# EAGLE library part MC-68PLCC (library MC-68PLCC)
SOCKET, PLCC, 68 PIN, THRU-HOLE Source: Datasheet
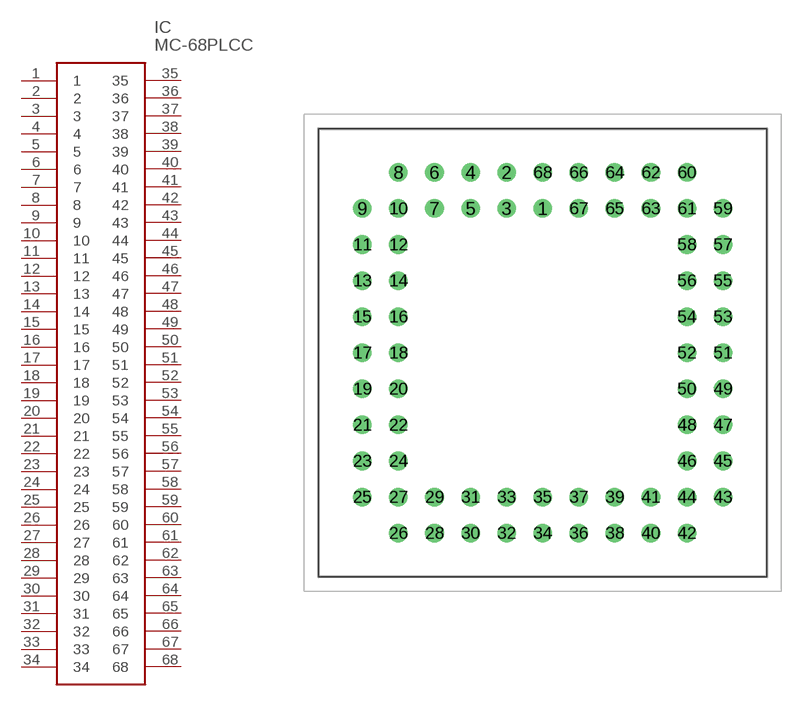
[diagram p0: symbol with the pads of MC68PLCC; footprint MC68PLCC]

Designator prefix IC

## MC-68PLCC (Description: SOCKET, PLCC, 68 PIN, THRU-HOLE; Height: 8.1mm; Manufacturer_Name: MULTICOMP; Manufacturer_Part_Number: MC-68PLCC)  [MC68PLCC]
1  1
2  2
3  3
4  4
5  5
6  6
7  7
8  8
9  9
10  10
11  11
12  12
13  13
14  14
15  15
16  16
17  17
18  18
19  19
20  20
21  21
22  22
23  23
24  24
25  25
26  26
27  27
28  28
29  29
30  30
31  31
32  32
33  33
34  34
35  35
36  36
37  37
38  38
39  39
40  40
41  41
42  42
43  43
44  44
45  45
46  46
47  47
48  48
49  49
50  50
51  51
52  52
53  53
54  54
55  55
56  56
57  57
58  58
59  59
60  60
61  61
62  62
63  63
64  64
65  65
66  66
67  67
68  68

## Footprint MC68PLCC (pad centres in mm)
MC-68PLCC-2
drill 0.8 pad 1.3: 1 0,0; 2 -2.54,2.54; 3 -2.54,0; 4 -5.08,2.54; 5 -5.08,0; 6 -7.62,2.54; 7 -7.62,0; 8 -10.16,2.54; 9 -12.7,0; 10 -10.16,0; 11 -12.7,-2.54; 12 -10.16,-2.54; 13 -12.7,-5.08; 14 -10.16,-5.08; 15 -12.7,-7.62; 16 -10.16,-7.62; 17 -12.7,-10.16; 18 -10.16,-10.16; 19 -12.7,-12.7; 20 -10.16,-12.7; 21 -12.7,-15.24; 22 -10.16,-15.24; 23 -12.7,-17.78; 24 -10.16,-17.78; 25 -12.7,-20.32; 26 -10.16,-22.86; 27 -10.16,-20.32; 28 -7.62,-22.86; 29 -7.62,-20.32; 30 -5.08,-22.86; 31 -5.08,-20.32; 32 -2.54,-22.86; 33 -2.54,-20.32; 34 0,-22.86; 35 0,-20.32; 36 2.54,-22.86; 37 2.54,-20.32; 38 5.08,-22.86; 39 5.08,-20.32; 40 7.62,-22.86; 41 7.62,-20.32; 42 10.16,-22.86; 43 12.7,-20.32; 44 10.16,-20.32; 45 12.7,-17.78; 46 10.16,-17.78; 47 12.7,-15.24; 48 10.16,-15.24; 49 12.7,-12.7; 50 10.16,-12.7; 51 12.7,-10.16; 52 10.16,-10.16; 53 12.7,-7.62; 54 10.16,-7.62; 55 12.7,-5.08; 56 10.16,-5.08; 57 12.7,-2.54; 58 10.16,-2.54; 59 12.7,0; 60 10.16,2.54; 61 10.16,0; 62 7.62,2.54; 63 7.62,0; 64 5.08,2.54; 65 5.08,0; 66 2.54,2.54; 67 2.54,0; 68 0,2.54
